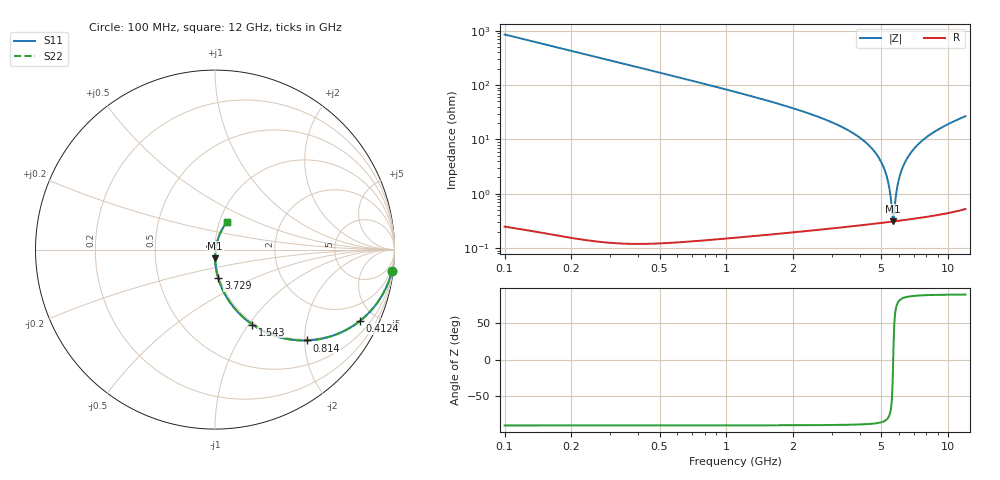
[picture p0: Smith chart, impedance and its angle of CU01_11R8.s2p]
! S-parameter model data by Modelithics Inc. support@modelithics.com 813-866-6335 Tampa FL USA
! S-Parameter data specifications:
! Substrate: 20-mil Rogers, substrate thickness, H=0.508mm, Dielectric constant, Er=3.75
! PCB Mounting Pad Footprint: Pad width, PadW=0.35mm , Pad length, PadL=0.30mm , Pad gap, PadG (edge-to-edge)=0.25mm , Reference planes=0.85mm apart
! Created Tue May  8 14:01:25 2018
# hz S ma R 50
! 2 Port Network Data from SP1.SP block
! freq  magS11  angS11  magS21  angS21  magS12  angS12  magS22  angS22
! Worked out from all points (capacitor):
!   801 points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, 100 MHz to 12 GHz, reference 50 ohm
!   read as one part in series: C = 1.86 pF near 159.5 MHz
!   lowest |Z| = 310 mohm at 5.663 GHz (marker M1)
!   series resonance near 5.669 GHz, so ESL is about 420 pH
!   S11 on the Smith chart (normalised r, x): 100 MHz: 1, -17; 412.4 MHz: 0.97, -4.08; 814 MHz: 0.97, -2.05; 1.543 GHz: 0.98, -1.04; 3.729 GHz: 0.98, -0.32; 12 GHz: 1.08, +0.34
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1e8  0.9932 -6.8  0.1158 83.2  0.1158 83.2  0.9932 -6.8
2.4875e8  0.9602 -16.4  0.2789 73.5  0.2789 73.5  0.9602 -16.4
4.12375e8  0.9004 -26.2  0.4345 63.8  0.4345 63.8  0.9004 -26.2
8.14e8  0.7201 -44.7  0.6929 45.3  0.6929 45.3  0.7201 -44.7
1.542875e9  0.4668 -63.5  0.8828 26.3  0.8828 26.3  0.4668 -63.5
2.09325e9  0.3487 -71.4  0.9354 18.3  0.9354 18.3  0.3487 -71.4
3.7295e9  0.1611 -83.5  0.9844 5.6  0.9844 5.6  0.1611 -83.5
4.071625e9  0.1364 -85.1  0.988 3.8  0.988 3.8  0.1364 -85.1
5.66325e9  0.04903 -89.2  0.9957 -2.8  0.9957 -2.8  0.04903 -89.2
6.05e9  0.03211 -88.5  0.9963 -4.1  0.9963 -4.1  0.03211 -88.5
6.481375e9  0.01461 -82.7  0.9965 -5.6  0.9965 -5.6  0.01461 -82.7
6.630125e9  0.009023 -74.6  0.9966 -6.1  0.9966 -6.1  0.009023 -74.6
6.79375e9  0.003951 -38.6  0.9965 -6.6  0.9965 -6.6  0.003951 -38.6
6.85325e9  0.003371 -4.0  0.9965 -6.8  0.9965 -6.8  0.003371 -4.0
6.91275e9  0.004153 28.5  0.9965 -7.0  0.9965 -7.0  0.004153 28.5
7.106125e9  0.01018 62.7  0.9964 -7.6  0.9964 -7.6  0.01018 62.7
7.2995e9  0.01697 70.0  0.9963 -8.2  0.9963 -8.2  0.01697 70.0
7.611875e9  0.02789 73.5  0.9959 -9.1  0.9959 -9.1  0.02789 73.5
8.04325e9  0.04257 74.6  0.9953 -10.4  0.9953 -10.4  0.04257 74.6
8.87625e9  0.06968 74.0  0.9935 -12.7  0.9935 -12.7  0.06968 74.0
1.002162e10  0.1051 71.7  0.99 -15.9  0.99 -15.9  0.1051 71.7
1.2e10  0.1642 66.9  0.9811 -21.3  0.9811 -21.3  0.1642 66.9
